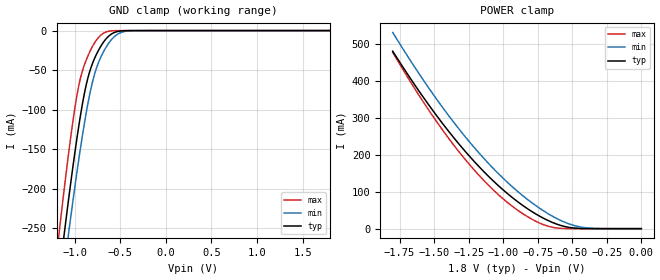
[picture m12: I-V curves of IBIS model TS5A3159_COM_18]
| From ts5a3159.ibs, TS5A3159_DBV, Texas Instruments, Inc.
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[Model]   TS5A3159_COM_18
Model_type  Terminator
| variable   typ   min   max
C_comp   47.59pF   39.75pF   52.40pF
| C_tri-state   47.59pF   39.75pF   52.40pF
[Temperature Range]   40   100   -40
| Ambient temperature   25   85   -40
[Voltage range]   1.8   1.65   1.95
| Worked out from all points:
|   GND clamp passes 1 mA (typ) near -0.52 V on its own axis
|   POWER clamp passes 1 mA (typ) near -0.46 V on its own axis
[GND Clamp]
| TS5A3159_COM_18
|   Voltage   I(typ)   I(min)   I(max)
-1.8V     -995.2mA   -1.009A    -986.8mA
-1.17V    -309mA     -349.9mA   -254.2mA
-1.115V   -256.8mA   -299mA     -199.8mA
-1.07V    -215.7mA   -258.7mA   -157.7mA
-990mV    -147.4mA   -190.5mA   -91.63mA
-925mV    -98.91mA   -139.6mA   -54.62mA
-870mV    -66.55mA   -101.3mA   -36.04mA
-805mV    -41.47mA   -64.93mA   -19.96mA
-685mV    -14.64mA   -26.79mA   -3.344mA
-555mV    -1.968mA   -6.643mA   -97.21uA
-410mV    -54.6uA    -466.8uA   -411.5nA
1.8V      2.505nA    7.567uA    1.919nA
[POWER Clamp]
| TS5A3159_COM_18
|   Voltage   I(typ)   I(min)   I(max)
-1.8V     480.3mA    531.1mA    477.3mA
-1.555V   343.2mA    389.3mA    329.6mA
-1.325V   231.2mA    272mA      210.3mA
-1.105V   141.1mA    175.9mA    117mA
-1V       104.7mA    136.2mA    80.53mA
-895mV    72.84mA    100.6mA    49.83mA
-785mV    44.55mA    68.02mA    24.22mA
-690mV    24.74mA    43.95mA    8.374mA
-590mV    9.47mA     23.32mA    1.099mA
-495mV    2.004mA    9.442mA    61.98uA
-355mV    65.8uA     963.5uA    302.6nA
0V        0A         0A         0A
